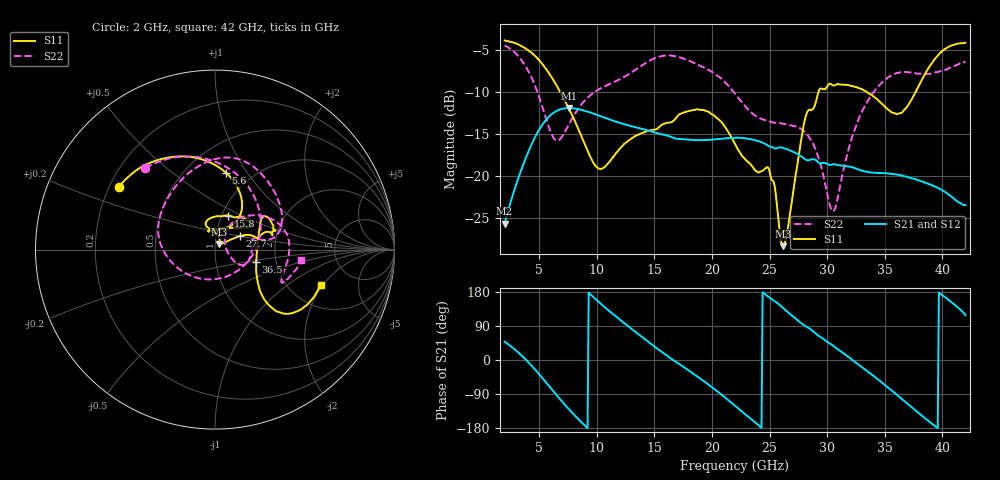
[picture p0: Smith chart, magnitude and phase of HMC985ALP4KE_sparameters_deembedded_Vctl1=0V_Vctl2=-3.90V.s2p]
!s2p File: Measurements: S11, S21, S12, S22
# GHz S dB R 50.0
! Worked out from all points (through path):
!   401 points, 2 GHz to 42 GHz, reference 50 ohm
!   highest |S21| = -11.93 dB at 7.6 GHz (marker M1); lowest = -25.7 dB at 2 GHz (marker M2)
!   lowest |S11| = -28.4 dB at 26.2 GHz (marker M3), VSWR 1.08, Z = 52.3 + j3.16 ohm
!   |S11| at or under -10 dB: 6.821 GHz to 29.25 GHz (22.43 GHz wide, 124 % of centre); 33.42 GHz to 37.69 GHz (4.271 GHz wide, 12 % of centre)
!   |S22| runs from -24.2 to -4.5 dB; largest |S21 - S12| = 0.0002
!   S11 on the Smith chart (normalised r, x): 2 GHz: 0.24, +0.28; 5.6 GHz: 0.76, +0.80; 15.8 GHz: 1.07, +0.42; 27.7 GHz: 1.30, +0.20; 36.5 GHz: 1.57, -0.23; 42 GHz: 2.94, -1.89
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2  -3.88 147.0  -25.69 48.5  -25.69 48.5  -4.47 130.6
3.6  -4.65 120.3  -18.72 8.2  -18.72 8.2  -6.49 85.1
4.6  -5.66 101.5  -15.51 -23.6  -15.51 -23.6  -9.12 48.0
5.6  -7.28 81.8  -13.32 -59.3  -13.33 -59.3  -13.18 -3.4
6.5  -9.22 66.5  -12.28 -92.2  -12.28 -92.3  -15.79 -69.4
7.6  -12.03 54.7  -11.93 -130.4  -11.93 -130.4  -13.82 -136.6
8.7  -15.38 54.9  -12.15 -165.0  -12.16 -165.0  -11.44 -170.9
10.4  -19.16 89.7  -12.93 147.1  -12.93 147.1  -9.54 161.8
15.4  -14.21 75.7  -14.99 27.0  -15.00 26.9  -5.82 86.3
15.8  -13.82 68.7  -15.09 18.0  -15.10 18.0  -5.70 81.3
19.3  -12.17 33.5  -15.73 -55.9  -15.74 -55.9  -7.09 35.7
22  -16.19 51.2  -15.46 -120.6  -15.46 -120.6  -10.21 10.4
24.9  -19.05 104.6  -16.44 166.8  -16.44 166.8  -13.49 13.0
26.2  -28.37 52.3  -16.68 136.5  -16.68 136.4  -13.81 -3.4
27.7  -16.12 28.6  -17.62 98.4  -17.63 98.3  -14.39 -24.2
28.7  -12.11 12.6  -18.02 77.8  -18.02 77.7  -15.95 -31.7
30.6  -9.26 19.6  -18.60 35.8  -18.61 35.8  -24.11 22.3
32.8  -9.58 33.9  -19.29 -14.1  -19.29 -14.1  -13.01 51.8
35.4  -12.22 11.7  -19.73 -75.5  -19.73 -75.5  -8.20 20.1
36.5  -12.47 -16.7  -19.96 -103.4  -19.97 -103.4  -7.64 6.3
39.5  -5.86 -43.7  -21.36 -177.3  -21.37 -177.4  -7.65 -25.9
42  -4.15 -18.6  -23.48 118.1  -23.49 118.1  -6.38 -6.7
